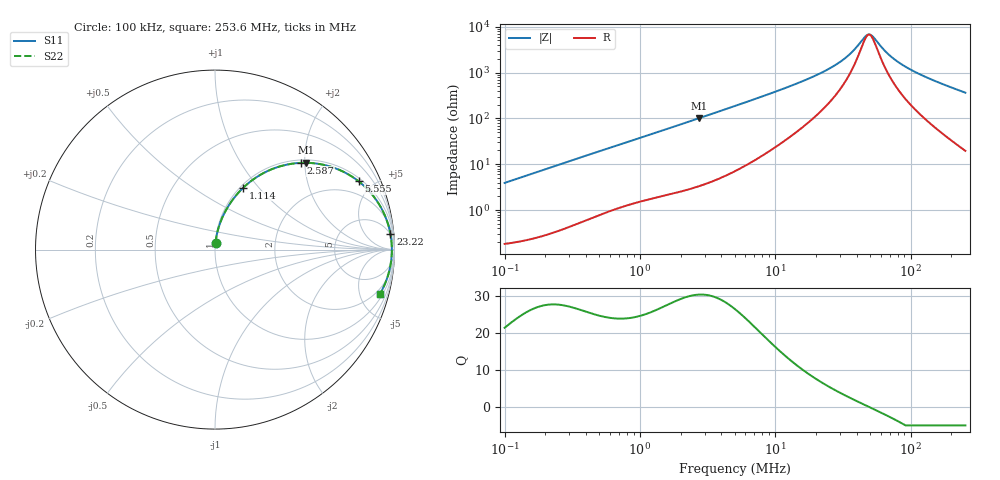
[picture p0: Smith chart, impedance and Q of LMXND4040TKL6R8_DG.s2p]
! LMXND4040TKL6R8_DG  S-PARAMETER MODEL  ( General Type )
! Model Generated by TAIYO YUDEN Corporation (http://www.ty-top.com)
! Version 1.0
! TAIYO YUDEN Control No. 191023NI43SB-FBB
! Copyright(c) 2019 TAIYO YUDEN CO.,LTD. All Rights Reserved.
! Product Description (link to TY-COMPAS)
! https://ds.yuden.co.jp/TYCOMPAS/or/detail?pn=LMXND4040TKL6R8MDG&u=M
! Products Name : Inductors
! Characteristics :
!  Inductance : 6.8 uH , SRF(min) : 30 MHz , DC Resistance(max) : 0.1176 Ohm
!  Rated Current : Saturation :1600 mA , Temp Rise : 1450 mA
!  Case Size : 4.0 x 4.0 / 0.157 x 0.157 [mm/inch] , Thickness : 1.8 / 0.071 [mm/inch]
!  (Conditions: Temperature = 25 degC , DC Bias Current/Voltage = 0A / 0V)
! External Node Assignments :
!  1  o---GGG---o  2
! GND o---------o GND
! Frequency Range : 0.1MHz  -  253.640152MHz  [ 402 STEP ]
# MHz S RI R 50
! Freq[MHz].  S11 Real  S11 Imag  S21 Real  S21 Imag  S12 Real  S12 Imag  S22 Real  S22 Imag
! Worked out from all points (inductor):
!   401 points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, 100 kHz to 253.6 MHz, reference 50 ohm
!   read as one part in series: L = 6.22 uH near 104 kHz
!   highest Q = 30.3 at 2.743 MHz (marker M1), where L = 5.88 uH
!   self-resonance near 49.24 MHz
!   S11 on the Smith chart (normalised r, x): 100 kHz: 1.00, +0.08; 1.114 MHz: 1.03, +0.83; 2.587 MHz: 1.06, +1.91; 5.555 MHz: 1.16, +4.13; 23.22 MHz: 4, +21; 253.6 MHz: 1.39, -7.26
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0.1  0.00335 0.039  0.9967 -0.039  0.9967 -0.039  0.00335 0.039
0.371712  0.0253 0.1392  0.9747 -0.1392  0.9747 -0.1392  0.0253 0.1392
0.682391  0.0717 0.238  0.9283 -0.238  0.9283 -0.238  0.0717 0.238
1.113774  0.1578 0.3452  0.8422 -0.3452  0.8422 -0.3452  0.1578 0.3452
1.381698  0.218 0.3945  0.782 -0.3945  0.782 -0.3945  0.218 0.3945
2.586726  0.4781 0.4833  0.5219 -0.4833  0.5219 -0.4833  0.4781 0.4833
2.743356  0.5064 0.4838  0.4936 -0.4838  0.4936 -0.4838  0.5064 0.4838
5.03627  0.7688 0.4031  0.2312 -0.4031  0.2312 -0.4031  0.7688 0.4031
5.554714  0.8005 0.3802  0.1995 -0.3802  0.1995 -0.3802  0.8005 0.3802
9.428583  0.9152 0.2508  0.0848 -0.2508  0.0848 -0.2508  0.9152 0.2508
18.72042  0.9705 0.1191  0.0295 -0.1191  0.0295 -0.1191  0.9705 0.1191
23.2237  0.9773 0.0879  0.0227 -0.0879  0.0227 -0.0879  0.9773 0.0879
33.70015  0.9836 0.0417  0.0164 -0.0417  0.0164 -0.0417  0.9836 0.0417
38.655  0.9847 0.0263  0.0153 -0.0263  0.0153 -0.0263  0.9847 0.0263
46.11058  0.9854 0.00707  0.0146 -0.00707  0.0146 -0.00707  0.9854 0.00707
48.90263  0.9855 0.000739  0.0145 -0.000739  0.0145 -0.000739  0.9855 0.000739
52.8901  0.9854 -0.0077  0.0146 0.0077  0.0146 0.0077  0.9854 -0.0077
69.58603  0.984 -0.0379  0.016 0.0379  0.016 0.0379  0.984 -0.0379
86.32529  0.9814 -0.0633  0.0186 0.0633  0.0186 0.0633  0.9814 -0.0633
113.5758  0.9753 -0.0997  0.0247 0.0997  0.0247 0.0997  0.9753 -0.0997
168.0725  0.9577 -0.1631  0.0423 0.1631  0.0423 0.1631  0.9577 -0.1631
253.6402  0.9182 -0.2484  0.0818 0.2484  0.0818 0.2484  0.9182 -0.2484
